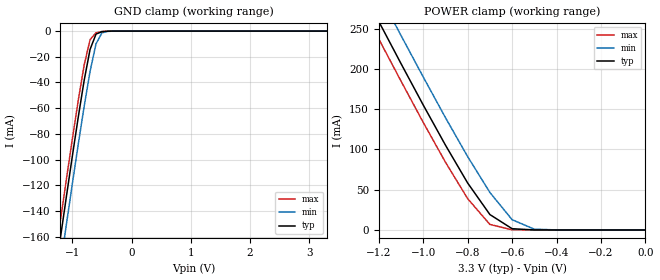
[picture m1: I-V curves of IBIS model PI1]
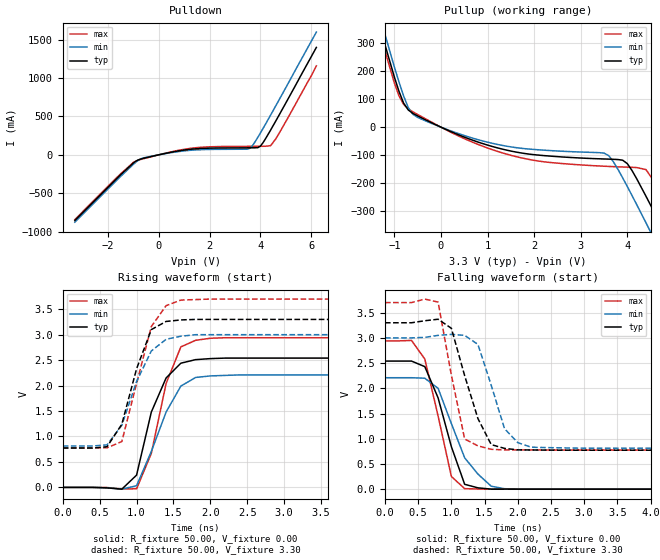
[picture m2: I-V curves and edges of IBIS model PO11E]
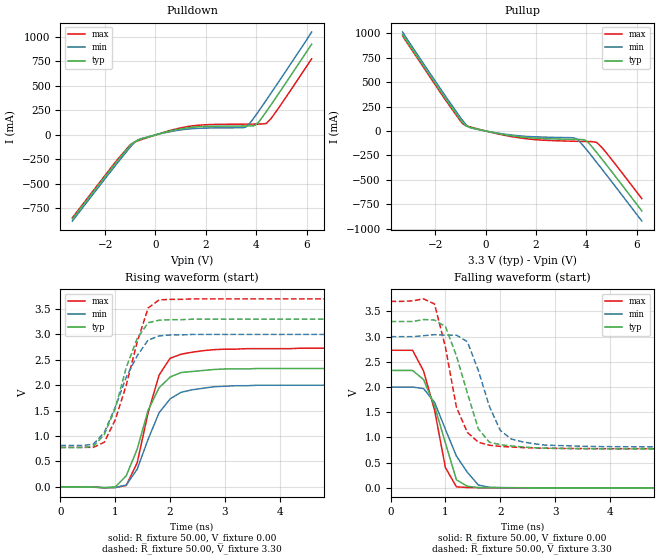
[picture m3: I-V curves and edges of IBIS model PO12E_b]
|   * 932s200.ibs * IBIS 2.1 Model file
| Rev History
| Rev No.   Description
| 1.0   Initial release with Updated Parasitic Parameters
| 1.1   ibis revisit
[IBIS Ver]   2.1
[Comment char]  |_char
[File name]   932s200.ibs
[Date]   August 29, 2002
[File Rev]   1.1
[Source]   Originated at Integrated Circuit Systems, Inc.
[Disclaimer] (C) Copyright Integrated Circuit Systems, Inc. 2002
   All rights reserved
ICS hereby grants the user of this IBIS model a non-exclusive,
nontransferable license to use this IBIS model under the following terms.
Before using this IBIS model, the user should read this license.
If the user does not accept these terms,  the IBIS model should be
returned to ICS within 30 days.
   The user is granted this license only to use the IBIS model and
is not granted rights to sell, load, rent, lease or license the IBIS
model in whole or in part, or in modified form to anyone other than
user. User may modify the IBIS model to suit its specific
applications but rights to derivative works and such modifications
shall belong to ICS.
   This IBIS model is provided on an "AS IS" basis and ICS makes
absolutely no warranty with respect to the information contained
herein. ICS DISCLAIMS AND CUSTOMER WAIVES ALL WARRANTIES, EXPRESS
OR IMPLIED, INCLUDING WARRANTIES OF MERCHANTABILITY OR FITNESS FOR
A PARTICULAR PURPOSE. The entire risk as to quality and performance
is with the Customer. ACCORDINGLY, IN NO EVENT SHALL THE COMPANY BE
LIABLE FOR ANY DAMAGES, WHETHER IN CONTRACT OR TORT,INCLUDING ANY
LOST PROFITS OR OTHER INCIDENTAL, CONSEQUENTIAL, EXEMPLARY, OR
PUNITIVE DAMAGES ARISING OUT OF THE USE OR APPLICATION OF THE IBIS
model provided in this package. Further, ICS reserves the right to
make changes without notice to any product herein to improve
reliability, function, or design. ICS does not convey any license
under patent rights or any other intellectual property rights,
including those of third parties.
   ICS is not obligated to provide maintenance or support
for the licensed IBIS model.
|   COMPONENT: ICS932s200
[Component]   ICS932s200
[Manufacturer]  ICS
[Package]
| variable   typ   min   max
R_pkg   81.1m   62.2m   100.0m
L_pkg   6.7nH   4.9nH   8.5nH
C_pkg   0.53pF  0.21pF  0.85pF
[Pin]   signal_name   model_name   R_pin   L_pin   C_pin
  1   GND   GND
  2   REF0   PO1E11
  3   REF1   PO1E11
  4   VDD   POWER
  5   X1   PXTAL1
  6   X2   PXTAL2
  7   GND   GND
  8   GND   GND
  9   PCICLK_F   PO11E
 10   VDD   POWER
 11   PCICLK0   PO11E
 12   PCICLK1   PO11E
 13   GND   GND
 14   PCICLK2   PO11E
 15   PCICLK3   PO11E
 16   VDD   POWER
 17   VDD   POWER
 18   PCICLK4   PO11E
 19   GND   GND
 20   GND   GND
 21   GND   GND
 22   VDD   POWER
 23   VDD   POWER
 24   GND   GND
 25   3V66_0   PO12E_b
 26   3V66_1   PO12E_b
 27   VDD   POWER
 28   SEL133/100#   PI1
 29   GND   GND
 30   48MHz   PO1E11
 31   VDD   POWER
 32   SEL0   PI1
 33   SEL1   PI1
 34   SPREAD#   PI1
 35   PD#   PI1
 36   CPU_STOP#   PI1
 37   PCI_STOP#   PI1
 38   GND   GND
 39   VDD   POWER
 40   GND   GND
 41   CPUCLK0   PO36L
 42   CPUCLK1   PO36L
 43   VDDL   POWER
 44   GND   GND
 45   CPUCLK2   PO36L
 46   CPUCLK3   PO36L
 47   VDDL   POWER
 48   GND   GND
 49   CPUCLK4   PO36L
 50   CPUCLK5   PO36L
 51   VDDL   POWER
 52   GND   GND
 53   IOAPIC0   PO22L
 54   IOAPIC1   PO22L
 55   IOAPIC2   PO22L
 56   VDDL   POWER
| Models and submodels in the file (8): PI1 (Input), PO11E (Output), PO12E_b (Output), PO1E11 (Output), PO22L (Output), PO36L (Output), PXTAL1 (Input), PXTAL2 (Input)
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|* Either 3.3V or 2.5V
|** All model are simulated with typical corner process
|   Model PI1
[Model]   PI1
Model_type   Input
Polarity   Non-Inverting
Vinl = 800.00mV
Vinh =   2.00V
C_comp   5.50pF   5.00pF   6.00pF
[Temperature Range]   27.00   70.00   0.00
[Voltage Range]   3.30V   3.00V   3.70V
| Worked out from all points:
|   GND clamp passes 1 mA (typ) near -0.53 V on its own axis
|   POWER clamp passes 1 mA (typ) near -0.56 V on its own axis
[GND_clamp]
| voltage   I(typ)   I(min)   I(max)
-3.3V     -857mA     -877.7mA   -844.3mA
-1.3V     -193.1mA   -214.7mA   -179.6mA
-1.2V     -160.8mA   -182.5mA   -147.3mA
-1.1V     -128.9mA   -150.6mA   -115.5mA
-1V       -97.6mA    -119.1mA   -84.25mA
-900mV    -67.14mA   -88.3mA    -54.11mA
-800mV    -38.43mA   -58.65mA   -26.49mA
-700mV    -14.23mA   -31.32mA   -6.64mA
-600mV    -2.36mA    -9.93mA    -1.32mA
-500mV    -489.3uA   -1.38mA    -326.7uA
-400mV    -91.06uA   -228.9uA   -44.42uA
3.3V      108.9pA    1.5uA      48.42pA
[POWER_clamp]
| voltage   I(typ)   I(min)   I(max)
-3.3V     1.4A       1.43A      1.38A
-1.3V     311.6mA    346.5mA    289.9mA
-1.2V     258.8mA    293.7mA    237mA
-1.1V     206.5mA    241.4mA    184.8mA
-1V       155.1mA    189.9mA    133.5mA
-900mV    105.3mA    139.4mA    84.13mA
-800mV    58.26mA    91.04mA    38.85mA
-700mV    19.13mA    46.53mA    6.83mA
-600mV    1.55mA     12.75mA    234.8uA
-500mV    47.55uA    992.2uA    4.48uA
-400mV    1.09uA     42uA       71.42nA
0V        108.9pA    1.22nA     66.46pA
|   Model PO11E
[Model]   PO11E
Model_type   Output
Polarity   Non-Inverting
|Vinl = 800.00mV
|Vinh =   2.00V
Vmeas =   1.50V
Cref =  30.00pF
Rref =  0.000
Vref =   1.50V
C_comp   5.50pF   5.00pF   6.00pF
[Temperature Range]   27.00   70.00   0.00
[Voltage Range]   3.30V   3.00V   3.70V
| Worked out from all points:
|   slope of the pulldown table from 0 to 0.495 V, typ, clamps not added: 14.5 ohm
|   slope of the pullup table from 0 to 0.495 V, typ, clamps not added: 14.1 ohm
|   rising waveform, R_fixture 50.00, V_fixture 0.00: 20-80 % time 322ps typ, 392ps min, 310ps max; typ from 0 V to 2.54 V
|   rising waveform, R_fixture 50.00, V_fixture 3.30: 20-80 % time 314ps typ, 354ps min, 311ps max; typ from 0.772 V to 3.3 V
|   falling waveform, R_fixture 50.00, V_fixture 0.00: 20-80 % time 361ps typ, 445ps min, 304ps max; typ from 2.54 V to 0 V
|   falling waveform, R_fixture 50.00, V_fixture 3.30: 20-80 % time 363ps typ, 312ps min, 260ps max; typ from 3.3 V to 0.772 V
[Pulldown]
| voltage   I(typ)   I(min)   I(max)
-3.3V     -857.8mA   -878.3mA   -845.1mA
-1.5V     -260.9mA   -281.8mA   -248.1mA
-1V       -106.4mA   -124.1mA   -99.56mA
-700mV    -54.41mA   -51.21mA   -59.61mA
300mV     21.43mA    18mA       24.36mA
1.3V      73.78mA    60.41mA    86.54mA
3.6V      91.32mA    88.09mA    110.4mA
3.9V      93.64mA    229.1mA    111mA
4V        113.7mA    285.1mA    111.2mA
4.4V      322mA      517.9mA    119.7mA
4.8V      557.1mA    756.3mA    317.8mA
6.2V      1.4A       1.6A       1.16A
[Pullup]
| voltage   I(typ)   I(min)   I(max)
-3.3V     1.55A      1.59A      1.53A
-1.5V     466mA      504mA      442.5mA
-900mV    128.1mA    161.6mA    111.6mA
-700mV    61.3mA     69.75mA    65.06mA
-500mV    40.14mA    34.9mA     45.21mA
1.5V      -85.24mA   -70.44mA   -100.4mA
3.5V      -113.6mA   -92.61mA   -139.4mA
4V        -130.2mA   -212mA     -142.8mA
4.4V      -246.3mA   -341.1mA   -151.4mA
4.8V      -376.8mA   -473.3mA   -261.9mA
5.2V      -509.8mA   -606.9mA   -392.6mA
6.2V      -846.3mA   -943.5mA   -727.9mA
[Ramp]
| variable   typ   min   max
dV/dt_r   1.53/245.67p   1.33/285.50p   1.77/205.68p
dV/dt_f   1.52/200.00p   1.31/300.00p   1.75/200.00p
[Rising Waveform]
R_fixture = 50.00
V_fixture = 0.00
V_fixture_min = 0.00
V_fixture_max = 0.00
| time   V(typ)   V(min)   V(max)
0s        0V         0V         0V
600ps     -9.4mV     -8.53mV    -2.42mV
800ps     -34.85mV   -34.36mV   -31.41mV
1ns       241mV      33.02mV    -27.25mV
1.2ns     1.48V      706.8mV    668.2mV
1.4ns     2.15V      1.48V      2.04V
1.6ns     2.44V      1.99V      2.76V
1.8ns     2.51V      2.16V      2.89V
2.2ns     2.54V      2.2V       2.94V
10ns      2.54V      2.21V      2.94V
[Rising Waveform]
R_fixture = 50.00
V_fixture = 3.30
V_fixture_min = 3.00
V_fixture_max = 3.70
| time   V(typ)   V(min)   V(max)
0s        772.3mV    812.8mV    776.4mV
400ps     772.1mV    812.5mV    776.3mV
600ps     799.2mV    835.8mV    777.7mV
800ps     1.24V      1.22V      900.5mV
1ns       2.33V      2.08V      2.04V
1.2ns     3.1V       2.68V      3.16V
1.4ns     3.26V      2.91V      3.57V
1.6ns     3.29V      2.97V      3.68V
1.8ns     3.3V       3V         3.69V
10ns      3.3V       3V         3.7V
[Falling Waveform]
R_fixture = 50.00
V_fixture = 0.00
V_fixture_min = 0.00
V_fixture_max = 0.00
| time   V(typ)   V(min)   V(max)
0s        2.54V      2.21V      2.94V
400ps     2.54V      2.21V      2.95V
600ps     2.43V      2.2V       2.58V
800ps     1.81V      2V         1.45V
1ns       842mV      1.3V       251.7mV
1.2ns     96.36mV    621.7mV    10.39mV
1.4ns     26.16mV    298.7mV    3.62mV
1.6ns     764.2uV    58.48mV    1.54mV
1.8ns     1.47mV     8.9mV      535uV
10ns      -3.88uV    -2.44uV    2.13uV
[Falling Waveform]
R_fixture = 50.00
V_fixture = 3.30
V_fixture_min = 3.00
V_fixture_max = 3.70
| time   V(typ)   V(min)   V(max)
0s        3.3V       3V         3.7V
800ps     3.37V      3.05V      3.71V
1ns       3.19V      3.07V      2.26V
1.2ns     2.25V      3.05V      994.7mV
1.4ns     1.4V       2.87V      858.5mV
1.6ns     883.5mV    2.06V      790.2mV
1.8ns     808.6mV    1.2V       778.6mV
2ns       779.4mV    922.5mV    778.6mV
2.2ns     776.8mV    832.1mV    777.6mV
10ns      772.3mV    812.8mV    776.4mV
|   Model PO12E_b
[Model]   PO12E_b
Model_type   Output
Polarity   Non-Inverting
|Vinl = 800.00mV
|Vinh =   2.00V
Vmeas =   1.50V
Cref =  30.00pF
Rref =  0.000
Vref =   1.50V
C_comp   5.50pF   5.00pF   6.00pF
[Temperature Range]   27.00   70.00   0.00
[Voltage Range]   3.30V   3.00V   3.70V
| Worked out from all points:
|   slope of the pulldown table from 0 to 0.495 V, typ, clamps not added: 14.5 ohm
|   slope of the pullup table from 0 to 0.495 V, typ, clamps not added: 18.8 ohm
|   rising waveform, R_fixture 50.00, V_fixture 0.00: 20-80 % time 466ps typ, 486ps min, 381ps max; typ from 0 V to 2.33 V
|   rising waveform, R_fixture 50.00, V_fixture 3.30: 20-80 % time 459ps typ, 520ps min, 467ps max; typ from 0.772 V to 3.3 V
|   falling waveform, R_fixture 50.00, V_fixture 0.00: 20-80 % time 406ps typ, 506ps min, 339ps max; typ from 2.33 V to 0 V
|   falling waveform, R_fixture 50.00, V_fixture 3.30: 20-80 % time 430ps typ, 436ps min, 371ps max; typ from 3.3 V to 0.772 V
[Pulldown]
| voltage   I(typ)   I(min)   I(max)
-3.3V     -857.8mA   -878.3mA   -845.1mA
-1.5V     -260.9mA   -281.8mA   -248.1mA
-1V       -106.4mA   -124.1mA   -99.56mA
-700mV    -54.41mA   -51.21mA   -59.61mA
300mV     21.43mA    18mA       24.36mA
1.3V      73.78mA    60.41mA    86.54mA
2.1V      87.67mA    70.65mA    105.3mA
3.6V      91.32mA    82.18mA    110.4mA
4V        105.2mA    207.1mA    111.2mA
4.4V      237.4mA    355.2mA    116.5mA
4.8V      387.1mA    507mA      242.1mA
6.2V      925.7mA    1.05A      776.2mA
[Pullup]
| voltage   I(typ)   I(min)   I(max)
-3.3V     983.7mA    1.01A      969.4mA
-1.5V     295.3mA    319.2mA    280.6mA
-900mV    81.81mA    102.4mA    72.29mA
-800mV    56.16mA    70.86mA    55.66mA
-600mV    36.42mA    32.43mA    40.85mA
500mV     -26.52mA   -22.39mA   -30.58mA
1.9V      -72.3mA    -58.7mA    -86.64mA
3.6V      -85.61mA   -78.64mA   -105.1mA
4V        -101.2mA   -188.8mA   -107.1mA
4.4V      -216.9mA   -317.6mA   -115.3mA
4.8V      -347.1mA   -449.6mA   -225.3mA
6.2V      -815.5mA   -918.7mA   -690mA
[Ramp]
| variable   typ   min   max
dV/dt_r   1.40/411.24p   1.20/464.87p   1.64/374.74p
dV/dt_f   1.52/300.00p   1.31/400.00p   1.75/300.00p
[Rising Waveform]
R_fixture = 50.00
V_fixture = 0.00
V_fixture_min = 0.00
V_fixture_max = 0.00
| time   V(typ)   V(min)   V(max)
0s        0V         0V         0V
1ns       -2.02mV    -13.17mV   -13.45mV
1.2ns     216.6mV    35.11mV    25.72mV
1.4ns     742.4mV    346.6mV    473.9mV
1.6ns     1.51V      937.9mV    1.46V
1.8ns     1.95V      1.46V      2.2V
2ns       2.16V      1.73V      2.53V
2.2ns     2.25V      1.86V      2.61V
3.6ns     2.33V      2V         2.72V
10ns      2.33V      2V         2.73V
[Rising Waveform]
R_fixture = 50.00
V_fixture = 3.30
V_fixture_min = 3.00
V_fixture_max = 3.70
| time   V(typ)   V(min)   V(max)
0s        772.3mV    812.8mV    776.4mV
600ps     795.5mV    838.9mV    777mV
800ps     1.03V      1.07V      877.7mV
1ns       1.54V      1.57V      1.32V
1.2ns     2.35V      2.16V      2V
1.4ns     2.92V      2.58V      2.85V
1.6ns     3.23V      2.89V      3.52V
1.8ns     3.28V      2.97V      3.68V
2.4ns     3.3V       3V         3.7V
10ns      3.3V       3V         3.7V
[Falling Waveform]
R_fixture = 50.00
V_fixture = 0.00
V_fixture_min = 0.00
V_fixture_max = 0.00
| time   V(typ)   V(min)   V(max)
0s        2.33V      2V         2.73V
400ps     2.33V      2V         2.73V
600ps     2.15V      1.97V      2.32V
800ps     1.63V      1.7V       1.55V
1ns       886.7mV    1.16V      399.8mV
1.2ns     160.8mV    630.1mV    20.36mV
1.4ns     30.45mV    308.3mV    7.05mV
1.6ns     6.18mV     57.3mV     3.64mV
1.8ns     3.79mV     11.46mV    2.58mV
10ns      0V         -2.85uV    -2.3uV
[Falling Waveform]
R_fixture = 50.00
V_fixture = 3.30
V_fixture_min = 3.00
V_fixture_max = 3.70
| time   V(typ)   V(min)   V(max)
0s        3.3V       3V         3.7V
800ps     3.33V      3.04V      3.65V
1ns       3.2V       3.03V      2.79V
1.2ns     2.62V      3.03V      1.6V
1.4ns     1.88V      2.9V       1.1V
1.6ns     1.17V      2.33V      904.9mV
1.8ns     905.8mV    1.62V      845.9mV
2.2ns     831.8mV    968.7mV    810.5mV
2.8ns     789.5mV    849.8mV    786.4mV
10ns      772.3mV    812.9mV    776.4mV
